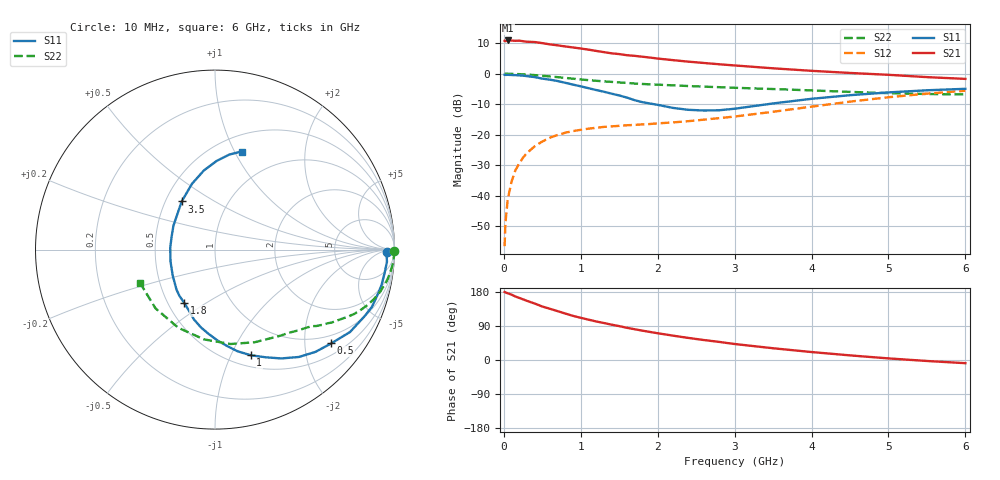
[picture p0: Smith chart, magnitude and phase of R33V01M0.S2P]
! SIEMENS Small Signal Semiconductors
! BFR181
! Si NPN RF Bipolar Junction Transistor in SOT23
! VCE = 3 V  IC = 1 mA
! Common Emitter S-Parameters:  May  1996
# GHz  S  MA  R  50
!  f  S11  S21  S12  S22
! GHz  MAG  ANG  MAG  ANG  MAG  ANG  MAG  ANG
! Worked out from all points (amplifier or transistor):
!   36 points, 10 MHz to 6 GHz, reference 50 ohm
!   highest |S21| = 10.9 dB at 50 MHz (marker M1)
!   |S21| within 3 dB of that: start of sweep to 1.098 GHz
!   unconditionally stable (mu >= 1): 2.017 GHz to 3.66 GHz
!   at 250 MHz: K = 0.15, MSG = 19.1 dB, |S12| = -27.5 dB
!   at 1.4 GHz: K = 0.77, MSG = 12.0 dB, |S12| = -17.2 dB
!   at 6 GHz: K = 0.88, MSG = 1.9 dB, |S12| = -5.6 dB
!   lowest NFmin = 1.30 dB at 450 MHz
!   S11 on the Smith chart (normalised r, x): 10 MHz: 43, -17; 500 MHz: 0.77, -2.63; 1 GHz: 0.62, -1.19; 1.8 GHz: 0.60, -0.41; 3.5 GHz: 0.60, +0.36; 6 GHz: 0.66, +1.07
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0.01  0.9606 -0.9  3.464 179.4  0.0015 92.3  0.9988 -0.4
0.02  0.9562 -1.4  3.411 178.3  0.0035 85.2  0.9992 -0.8
0.05  0.9605 -4.1  3.507 176.1  0.0087 87.4  0.9977 -1.9
0.1  0.9539 -7.9  3.492 172.5  0.0171 83.9  0.9962 -3.7
0.15  0.9485 -12.1  3.462 167.6  0.0262 81.6  0.9903 -5.6
0.2  0.9393 -15.8  3.48 163.9  0.034 79.6  0.9847 -7.4
0.3  0.9134 -23.8  3.344 156.1  0.0502 75.0  0.9701 -10.9
0.4  0.8814 -31.4  3.305 149.1  0.0646 70.1  0.95 -14.3
0.5  0.8321 -38.9  3.171 141.1  0.0776 65.9  0.9266 -17.4
0.7  0.7592 -52.0  2.915 128.8  0.0994 58.7  0.8787 -22.5
0.9  0.6631 -64.8  2.694 116.4  0.1151 52.7  0.8292 -26.8
1  0.6215 -71.3  2.588 111.3  0.1206 50.6  0.8052 -28.6
1.1  0.5802 -77.5  2.481 106.5  0.1259 48.8  0.785 -30.3
1.4  0.4718 -94.2  2.159 93.3  0.1375 44.9  0.7354 -34.7
1.8  0.3426 -120.1  1.9 77.5  0.1481 44.1  0.6803 -39.2
2.2  0.2755 -149.0  1.669 64.2  0.1596 45.2  0.6452 -44.3
2.6  0.2498 177.9  1.5 52.7  0.1769 48.0  0.6142 -49.6
3  0.2672 150.1  1.367 42.2  0.1991 50.3  0.5889 -56.2
3.5  0.3262 124.7  1.227 31.0  0.2382 51.5  0.5616 -66.8
4.5  0.4453 98.0  1.03 12.2  0.3491 47.1  0.5041 -96.9
5.5  0.5357 81.4  0.88 -2.6  0.4721 34.7  0.4658 -135.4
6  0.5666 74.7  0.823 -8.4  0.5273 26.8  0.4568 -155.7
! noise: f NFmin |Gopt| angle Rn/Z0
0.45  1.3  0.7  18  0.5
0.9  1.4  0.6  39  0.52
1.8  1.85  0.4  81  0.47
